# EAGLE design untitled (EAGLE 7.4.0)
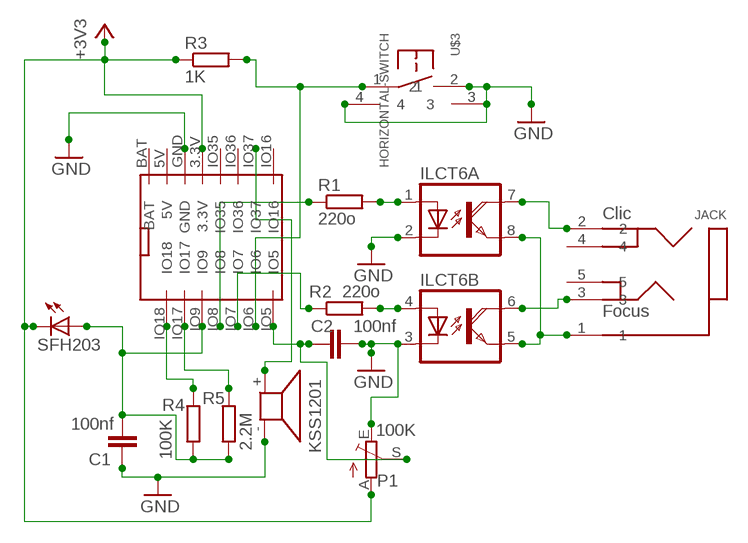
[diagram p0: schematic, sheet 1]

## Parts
C1  100nf  C-EU050-025X075  [C050-025X075]
C2  100nf  C-EU050-025X075  [C050-025X075]
ILCT6  ILD30  [DIL08]
JACK  JACK  [JACK2]
KSS1201  KSS1201  [KSS1201]
P1  100K  TRIM_EU-RJ9W  [RJ9W]
R1  220o  R-EU_0207/2V  [0207/2V]
R2  220o  R-EU_0207/2V  [0207/2V]
R3  1K  R-EU_0207/2V  [0207/2V]
R4  100K  R-EU_0207/2V  [0207/2V]
R5  2.2M  R-EU_0207/2V  [0207/2V]
SFH203  SFH203  [SFH203]
U$2  01SPACE-ESP32S3  [01SPACE-ESP32S3]
U$3  HORIZONTAL-SWITCH  [HORIZONTAL-SWITCH]

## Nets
+3V3: P1.A R3.1 SFH203.K(C) U$2.3.3V
GND: C1.2 C2.2 ILCT6.2(A:C) ILCT6.3(B:C) KSS1201.- P1.E U$2.GND U$3.2 U$3.3 U$3.4
N$1: C1.1 R4.1 R5.1 SFH203.A U$2.IO9
N$2: R4.2 U$2.IO18
N$3: R5.2 U$2.IO17
N$4: R3.2 U$2.IO6 U$3.1
N$6: KSS1201.+ U$2.IO37
N$7: C2.1 P1.S U$2.IO5
N$9: ILCT6.1(A:A) R1.2
N$10: ILCT6.4(B:A) R2.2
N$11: R1.1 U$2.IO8
N$12: R2.1 U$2.IO7
N$13: ILCT6.5(B:EMI) ILCT6.8(A:EMI) JACK.1
N$14: ILCT6.7(A:COL) JACK.2
N$15: ILCT6.6(B:COL) JACK.3
Unconnected: JACK.4 JACK.5 U$2.5V U$2.BAT U$2.IO16 U$2.IO35 U$2.IO36

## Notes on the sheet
- Clic
- Focus

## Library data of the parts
C1 C2 = resistor:C-EU: CAPACITOR, European symbol
ILCT6 = optocoupler:ILD30: SIEMENS OPTO COUPLER; MF: VISHAY/TELEFUNKEN; MPN: ILD30; OC_FARNELL: 1612448; OC_NEWARK: 58K1668
JACK = perso:JACK: PCB Stereo Jack 3.5mm
KSS1201 = buzzer:KSS1201: SPEAKER; OC_FARNELL: unknown; OC_NEWARK: unknown
P1 = pot:TRIM_EU-: POTENTIOMETER
R1-R5 = resistor:R-EU_: RESISTOR, European symbol
SFH203 = perso:SFH203
U$2 = perso:01SPACE-ESP32S3
U$3 = perso:HORIZONTAL-SWITCH

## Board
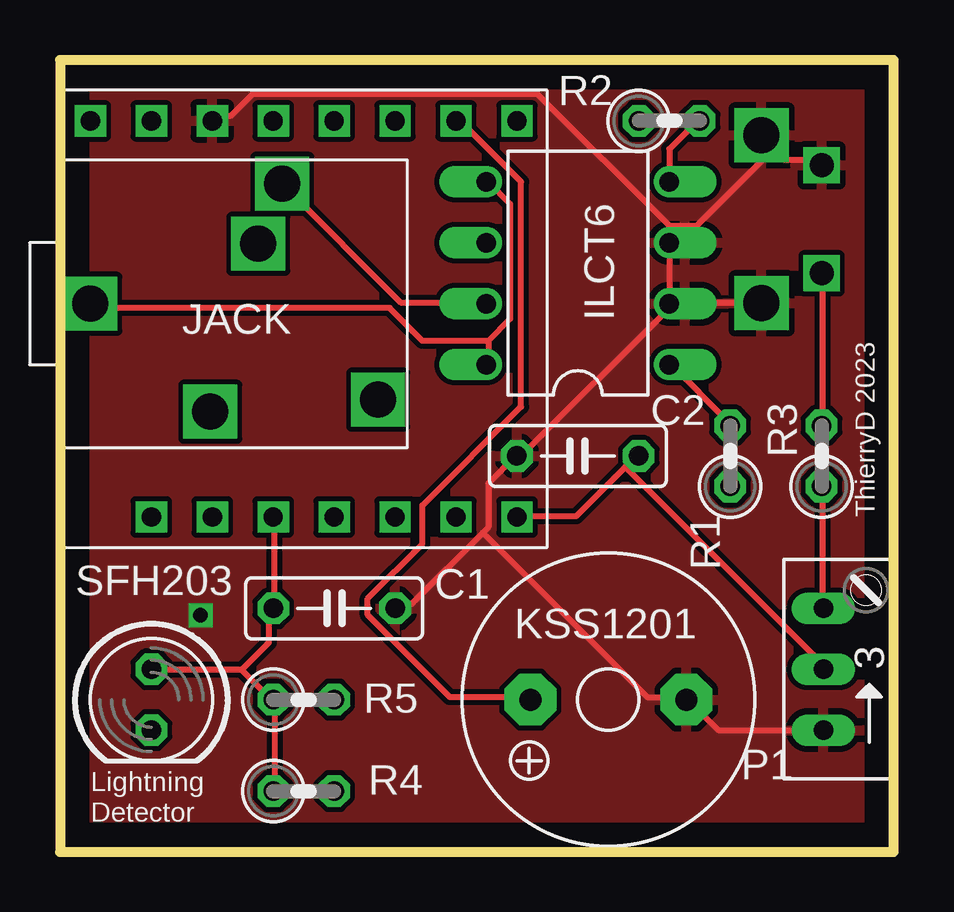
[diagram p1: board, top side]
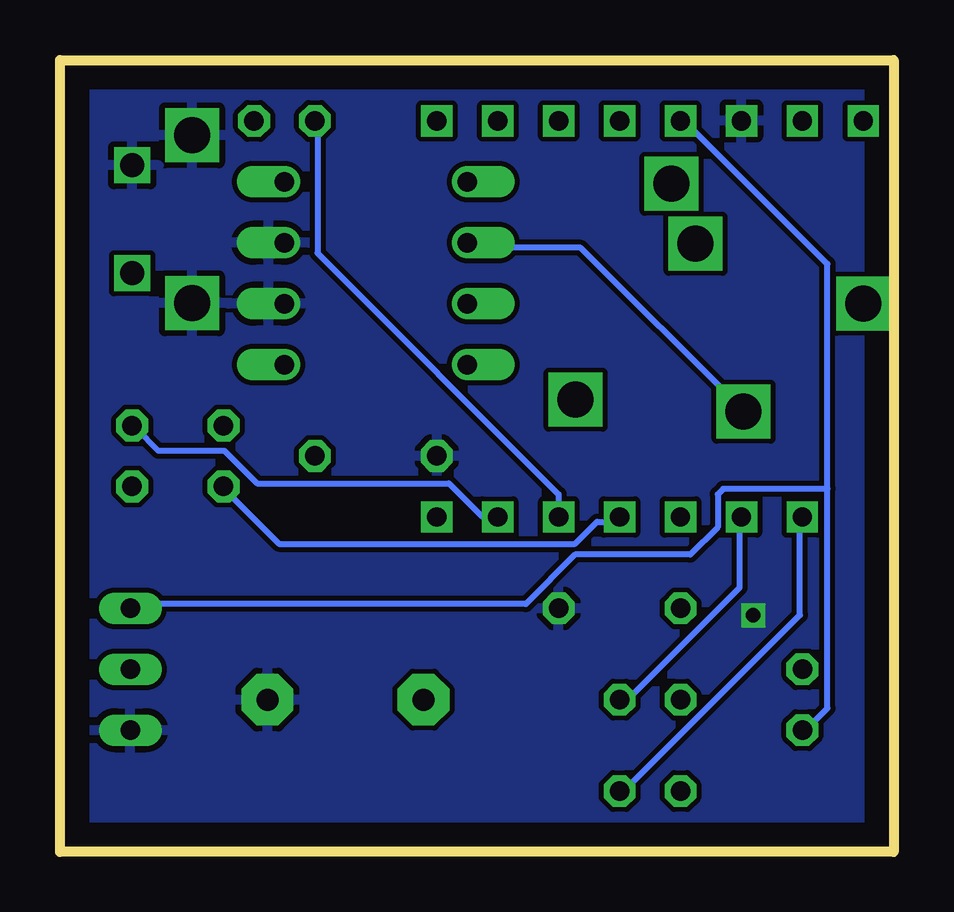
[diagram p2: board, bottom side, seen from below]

Size 34.76 x 33.02 mm. Coordinates in mm from the lower left corner, seen from the top.
Outline: 0,33.02 0,0 34.76,0 34.76,33.02 0,33.02
Copper layers (1*16): Top 0.035mm / dielectric 1.5mm / Bottom 0.035mm
Design rules "default": minimum track width 10mil, minimum drill 24mil, track to track 8mil, track to pad 8mil, pad to pad 8mil, via to via 8mil, smd to smd 8mil, copper to edge 40mil, drill to drill 8mil, minimum pad ring 10mil, minimum via ring 8mil, stop-mask expansion 4mil, vias tented up to drill 0mil, thermal gap 10mil

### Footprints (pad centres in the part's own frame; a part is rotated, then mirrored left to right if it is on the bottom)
C050-025X075 = drill 0.813 octagon: 1 -2.54,0; 2 2.54,0
DIL08 = drill 0.813 offset: 1 -3.81,-3.81; 2 -1.27,-3.81; 3 1.27,-3.81; 4 3.81,-3.81; 5 3.81,3.81; 6 1.27,3.81; 7 -1.27,3.81; 8 -3.81,3.81
JACK2 = drill 1.5 pad 2.184 square: 1 0,0; 2 8,5; 3 5,-4.5; 4 7,2.5; 5 12,-4
KSS1201 = drill 0.914 pad 2.159 octagon: + 3.251,0; - -3.251,0
RJ9W = drill 0.813 long: A 2.54,0.635; E -2.54,0.635; S 0,0.635
0207/2V = drill 0.813 octagon: 1 -1.27,0; 2 1.27,0
SFH203 = drill 0.813 octagon: A -1.27,0; K 1.27,0
01SPACE-ESP32S3 = drill 0.8 square: 3.3V 5.08,0; 5V 5.08,5.08; BAT 5.08,7.62; GND 5.08,2.54; IO5 -11.43,-10.16; IO6 -11.43,-7.62; IO7 -11.43,-5.08; IO8 -11.43,-2.54; IO9 -11.43,0; IO16 5.08,-10.16; IO17 -11.43,2.54; IO18 -11.43,5.08; IO35 5.08,-2.54; IO36 5.08,-5.08; IO37 5.08,-7.62
HORIZONTAL-SWITCH = drill 1 square: 1 0,0; 2 4.5,0 | drill 1.5 square: 3 -1.25,2.5; 4 5.75,2.5

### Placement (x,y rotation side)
C1  11.43,10.16 0 top
C2  21.59,16.51 180 top
ILCT6  21.59,24.13 90 top
JACK  1.27,22.86 0 top
KSS1201  22.86,6.35 180 top
P1  32.46,7.62 90 top
R1  27.94,16.51 90 top
R2  25.4,30.48 0 top
R3  31.75,16.51 90 top
R4  10.16,2.54 0 top
R5  10.16,6.35 0 top
SFH203  3.81,6.35 270 top
U$2  8.89,25.4 90 top
U$3  31.75,24.13 90 top

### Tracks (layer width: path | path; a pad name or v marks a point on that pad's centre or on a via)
+3V3
  Top 0.254: R3.1 31.8,15.14 31.8,10.34 P1.A
  Bottom 0.254: 2.77,15.14 2.77,5.99 3.68,5.08 SFH203.K | 2.77,15.14 2.77,24.51 8.71,30.45 U$2.3.3V | 2.77,15.14 7.11,15.14 7.34,14.91 7.34,13.54 8.48,12.39 13.28,12.39 15.34,10.34 31.8,10.34 P1.A
GND  (via drill 0.6)
  Top 0.254: P1.E 27.46,5.08 26.31,6.22 KSS1201.- 26.09,6.45 24.49,6.45 17.63,13.31 | 17.63,13.31 17.86,13.54 17.86,15.37 19,16.51 C2.2 19.23,16.51 25.4,22.68 ILCT6.2 25.4,22.91 | 17.63,13.31 14.66,10.34 13.97,10.34 C1.2 | 29.74,29.31 29.29,29.77 U$3.4 29.74,29.31 | 29.74,29.31 30.2,28.85 31.57,28.85 U$3.2 | 25.4,26.11 19.91,31.6 8.03,31.6 7.11,30.68 6.43,30.68 U$2.GND | 25.4,26.11 ILCT6.3 25.4,22.91 | 25.4,22.91 29.06,22.91 U$3.3 | 29.74,29.31 26.54,26.11 25.4,26.11
  other vias: 5.86,9.87
  pour Top: 0,33.02 35.56,33.02 35.56,0 0,0
  pour Bottom: 0,33.02 35.56,33.02 35.56,0 0,0
N$1
  Top 0.254: U$2.IO9 8.94,13.77 8.94,10.34 C1.1 8.71,10.11 8.71,8.74 7.57,7.59 | R4.1 8.94,2.56 8.94,6.22 R5.1 8.71,6.45 7.57,7.59 | 7.57,7.59 3.91,7.59 SFH203.A
N$2
  Bottom 0.254: U$2.IO18 3.91,13.77 3.91,9.88 11.23,2.56 R4.2
N$3
  Bottom 0.254: U$2.IO17 6.43,13.77 6.43,11.02 11.23,6.22 R5.2
N$4
  Top 0.254: U$3.1 31.8,24.05 31.8,17.88 R3.2
  Bottom 0.254: U$2.IO6 16.71,13.99 17.17,13.99 18.54,15.37 26.54,15.37 27.91,16.74 30.66,16.74 31.57,17.65 R3.2
N$6
  Top 0.254: U$2.IO37 16.71,30.45 19.23,27.94 19.23,18.57 15.11,14.45 15.11,12.85 12.83,10.57 12.83,9.88 16.26,6.45 19.46,6.45 KSS1201.+
N$7
  Top 0.254: 23.57,16.05 24.03,16.51 C2.1 | 23.57,16.05 21.51,13.99 19.23,13.99 U$2.IO5 | 23.57,16.05 31.8,7.82 P1.S
N$9
  Top 0.254: R1.2 27.91,17.88 25.4,20.4 ILCT6.1
N$10
  Top 0.254: ILCT6.4 25.4,29.31 26.54,30.45 R2.2
N$11
  Bottom 0.254: U$2.IO8 11.45,13.77 12.37,13.77 13.28,12.85 25.63,12.85 27.91,15.14 R1.1
N$12
  Bottom 0.254: U$2.IO7 13.97,14.91 24.03,24.97 24.03,30.45 R2.1
N$13
  Top 0.254: 17.86,21.31 17.86,20.4 ILCT6.8 | 17.86,21.31 18.77,22.22 18.77,27.03 17.86,27.94 ILCT6.5 | 17.86,21.31 15.11,21.31 13.74,22.68 1.4,22.68 JACK.1
N$14
  Top 0.254: ILCT6.7 17.63,22.91 14.2,22.91 9.4,27.71 JACK.2
N$15
  Bottom 0.254: ILCT6.6 17.63,25.2 13.06,25.2 6.43,18.57 JACK.3

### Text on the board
tNames: ThierryD 2023 | Lightning | Detector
